VAR_GLOBAL CONSTANT
	// constant for input
	cOversamples 	: UDINT 	:= 10;		// number of oversamples
	cFSample        : UDINT     := 10000;   // 1ms task with 10 oversamples = 10kHz
	
	// constants for FFT (Magnitude Spectrum)
	cBufferLength	: UDINT		:= 3200;	         // buffer size
	cWindowLength	: UDINT		:= 2*cBufferLength;	 // 50% overlap
	cFFTLength		: UDINT		:= 8192;	         // length of FFT for mag. spectrum, power of 2
	cFFTResult 		: UDINT 	:= cFFTLength/2+1;	 // result of mag. spectrum 
	
	// constant for averaging
	cNumAverage     : UDINT     := 25; 
	
	// number of classes for discrete classifictaion
	cMaxClasses : UDINT := 1;
	
	
	cThresholdBroadband	 : LREAL := 2;  // Thresold for classifier for all frequencies
	cThreshold50Hz	     : LREAL := 6;	// Thresold for classifier for a window from approx. 36 Hz to 61 Hz
END_VAR
